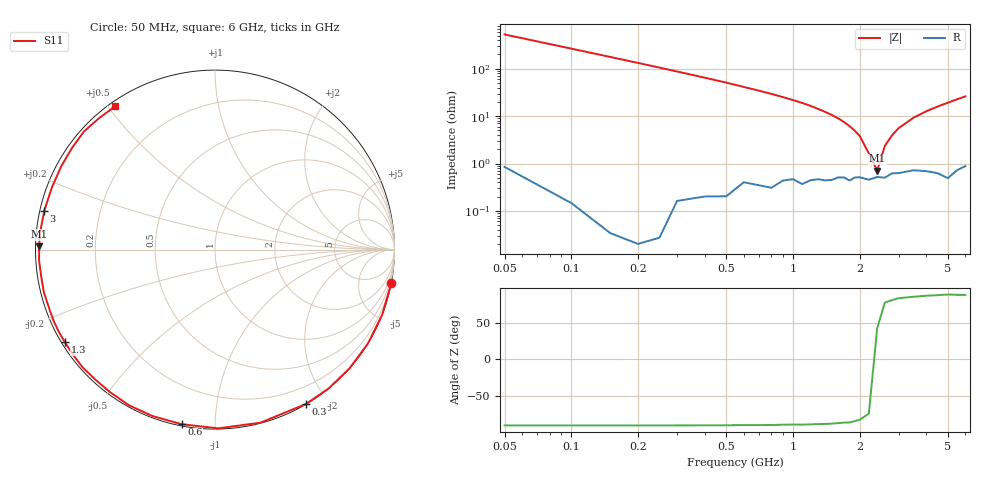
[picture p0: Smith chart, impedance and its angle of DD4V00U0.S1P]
! Infineon Technologies  Discrete & RF Semiconductors
! BBY58-02W
! Si Tuning Diode in SCD-80
! VR = 4 V
! S-Parameters:  June  2000
# GHz  S  MA  R  50
!  f  S11
! GHz  MAG  ANG
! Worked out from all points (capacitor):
!   34 points, 50 MHz to 6 GHz, reference 50 ohm
!   read as one part to ground: C = 5.97 pF near 50 MHz
!   lowest |Z| = 708 mohm at 2.4 GHz (marker M1)
!   series resonance near 2.353 GHz, so ESL is about 770 pH
!   S11 on the Smith chart (normalised r, x): 50 MHz: 0, -11; 300 MHz: 0.00, -1.75; 600 MHz: 0.01, -0.83; 1.3 GHz: 0.01, -0.28; 3 GHz: 0.01, +0.11; 6 GHz: 0.02, +0.52
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0.05  0.9997 -10.8
0.1  0.9998 -21.3
0.15  0.9999 -31.5
0.2  0.9999 -41.3
0.25  0.9998 -50.7
0.3  0.9984 -59.5
0.4  0.997 -75.3
0.5  0.996 -89.0
0.6  0.9905 -100.8
0.7  0.9906 -110.6
0.8  0.9909 -119.0
0.9  0.9862 -126.4
1  0.9844 -132.8
1.1  0.9872 -138.4
1.3  0.9829 -148.3
1.4  0.9835 -152.5
1.6  0.9805 -159.7
1.8  0.9829 -166.0
1.9  0.9801 -168.8
2.2  0.982 -176.4
2.4  0.9794 178.9
2.6  0.9801 174.7
3  0.9755 167.3
3.5  0.9725 159.1
4  0.9744 151.5
5  0.983 137.9
5.5  0.9763 131.3
6  0.9727 124.9
